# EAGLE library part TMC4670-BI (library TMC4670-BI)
Field oriented servocontrolerfor torque control,velocity control,and positioning. Encoder Engine, PWM-Engine und SPI. BGA256(17x17)
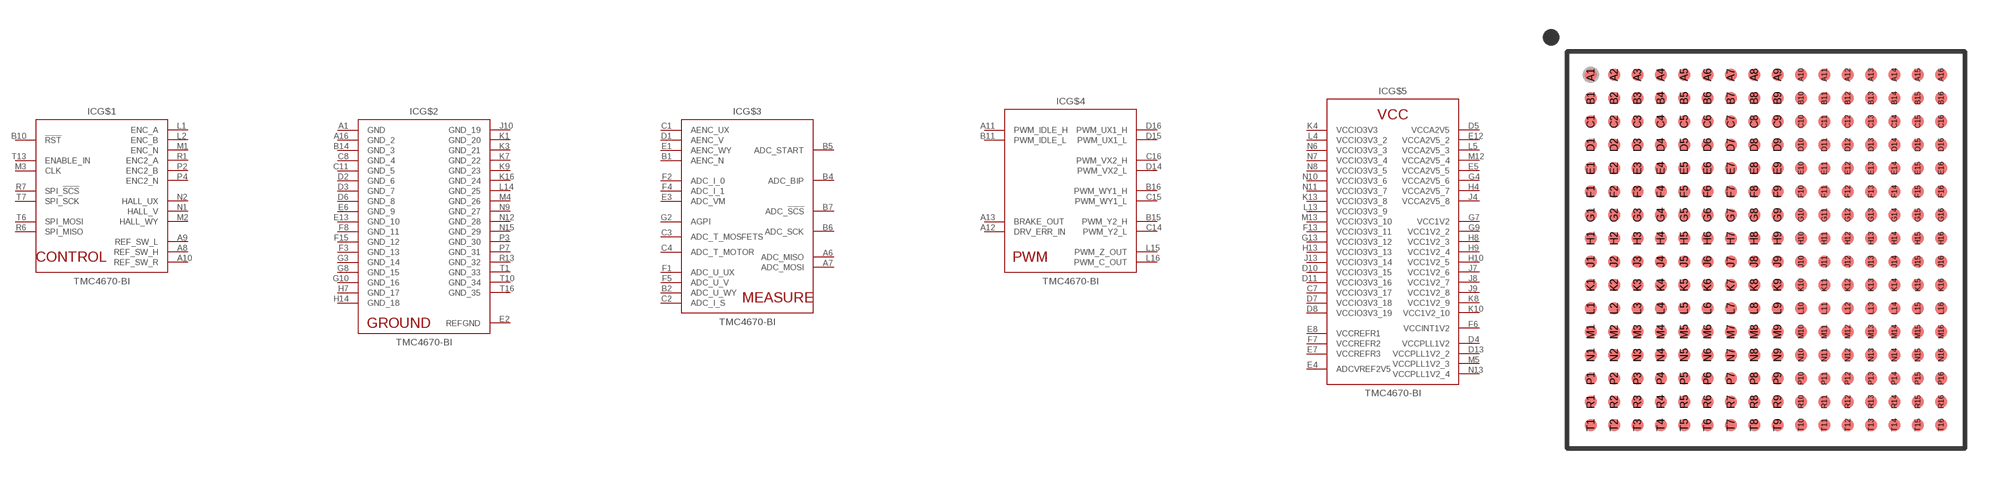
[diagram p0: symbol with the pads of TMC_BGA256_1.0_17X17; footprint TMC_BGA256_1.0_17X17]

Designator prefix IC; gates G$1=TMC4670_CONTROL G$2=TMC4670_GND G$3=TMC4670_MEASURE G$4=TMC4670_PWM G$5=TMC4670_VCC

## TMC4670-BI (DATASHEET: http://www.trinamic.com/fileadmin/assets/Products/ICs_Documents/tmc4670_datasheet.pdf; DESCRIPTION: Field oriented servocontrolerfor torque control,velocity control,and positioning_ Encoder Engine, PWM-Engine und SPI_ BGA256(17x17); GEOMETRY_HEIGHT: 2.2mm; MANUFACTURER: TRINAMIC; ORDERCODE-MANU1: TMC4670-BI; VALUE: TMC4670-BI)  [TMC_BGA256_1.0_17X17]
A1  G$2:GND  pwr
A6  G$3:ADC_MISO  out
A7  G$3:ADC_MOSI  out
A8  G$1:REF_SW_H  in
A9  G$1:REF_SW_L  in
A10  G$1:REF_SW_R  in
A11  G$4:PWM_IDLE_H  in
A12  G$4:DRV_ERR_IN  in
A13  G$4:BRAKE_OUT  out
A16  G$2:GND_2  pwr
B1  G$3:AENC_N  in
B2  G$3:ADC_U_WY  in
B4  G$3:ADC_BIP  out
B5  G$3:ADC_START  out
B6  G$3:ADC_SCK  out
B7  G$3:ADC_!SCS!  out
B10  G$1:!RST!  in
B11  G$4:PWM_IDLE_L  in
B14  G$2:GND_3  pwr
B15  G$4:PWM_Y2_H  out
B16  G$4:PWM_WY1_H  out
C1  G$3:AENC_UX  in
C2  G$3:ADC_I_S  in
C3  G$3:ADC_T_MOSFETS  in
C4  G$3:ADC_T_MOTOR  in
C7  G$5:VCCIO3V3_17  pwr
C8  G$2:GND_4  pwr
C11  G$2:GND_5  pwr
C14  G$4:PWM_Y2_L  out
C15  G$4:PWM_WY1_L  out
C16  G$4:PWM_VX2_H  out
D1  G$3:AENC_V  in
D2  G$2:GND_6  pwr
D3  G$2:GND_7  pwr
D4  G$5:VCCPLL1V2  pwr
D5  G$5:VCCA2V5  pwr
D6  G$2:GND_8  pwr
D7  G$5:VCCIO3V3_18  pwr
D8  G$5:VCCIO3V3_19  pwr
D10  G$5:VCCIO3V3_15  pwr
D11  G$5:VCCIO3V3_16  pwr
D13  G$5:VCCPLL1V2_2  pwr
D14  G$4:PWM_VX2_L  out
D15  G$4:PWM_UX1_L  out
D16  G$4:PWM_UX1_H  out
E1  G$3:AENC_WY  in
E2  G$2:REFGND  pwr
E3  G$3:ADC_VM  in
E4  G$5:ADCVREF2V5  pwr
E5  G$5:VCCA2V5_5  pwr
E6  G$2:GND_9  pwr
E7  G$5:VCCREFR3  pwr
E8  G$5:VCCREFR1  pwr
E12  G$5:VCCA2V5_2  pwr
E13  G$2:GND_10  pwr
F1  G$3:ADC_U_UX  in
F2  G$3:ADC_I_0  in
F3  G$2:GND_13  pwr
F4  G$3:ADC_I_1  in
F5  G$3:ADC_U_V  in
F6  G$5:VCCINT1V2  pwr
F7  G$5:VCCREFR2  pwr
F8  G$2:GND_11  pwr
F13  G$5:VCCIO3V3_11  pwr
F15  G$2:GND_12  pwr
G2  G$3:AGPI  in
G3  G$2:GND_14  pwr
G4  G$5:VCCA2V5_6  pwr
G7  G$5:VCC1V2  pwr
G8  G$2:GND_15  pwr
G9  G$5:VCC1V2_2  pwr
G10  G$2:GND_16  pwr
G13  G$5:VCCIO3V3_12  pwr
H4  G$5:VCCA2V5_7  pwr
H7  G$2:GND_17  pwr
H8  G$5:VCC1V2_3  pwr
H9  G$5:VCC1V2_4  pwr
H10  G$5:VCC1V2_5  pwr
H13  G$5:VCCIO3V3_13  pwr
H14  G$2:GND_18  pwr
J4  G$5:VCCA2V5_8  pwr
J7  G$5:VCC1V2_6  pwr
J8  G$5:VCC1V2_7  pwr
J9  G$5:VCC1V2_8  pwr
J10  G$2:GND_19  pwr
J13  G$5:VCCIO3V3_14  pwr
K1  G$2:GND_20  pwr
K3  G$2:GND_21  pwr
K4  G$5:VCCIO3V3  pwr
K7  G$2:GND_22  pwr
K8  G$5:VCC1V2_9  pwr
K9  G$2:GND_23  pwr
K10  G$5:VCC1V2_10  pwr
K13  G$5:VCCIO3V3_8  pwr
K16  G$2:GND_24  pwr
L1  G$1:ENC_A  in
L2  G$1:ENC_B  in
L4  G$5:VCCIO3V3_2  pwr
L5  G$5:VCCA2V5_3  pwr
L13  G$5:VCCIO3V3_9  pwr
L14  G$2:GND_25  pwr
L15  G$4:PWM_Z_OUT  out
L16  G$4:PWM_C_OUT  out
M1  G$1:ENC_N  in
M2  G$1:HALL_WY  in
M3  G$1:CLK  in
M4  G$2:GND_26  pwr
M5  G$5:VCCPLL1V2_3  pwr
M12  G$5:VCCA2V5_4  pwr
M13  G$5:VCCIO3V3_10  pwr
N1  G$1:HALL_V  in
N2  G$1:HALL_UX  in
N6  G$5:VCCIO3V3_3  pwr
N7  G$5:VCCIO3V3_4  pwr
N8  G$5:VCCIO3V3_5  pwr
N9  G$2:GND_27  pwr
N10  G$5:VCCIO3V3_6  pwr
N11  G$5:VCCIO3V3_7  pwr
N12  G$2:GND_28  pwr
N13  G$5:VCCPLL1V2_4  pwr
N15  G$2:GND_29  pwr
P2  G$1:ENC2_B  in
P3  G$2:GND_30  pwr
P4  G$1:ENC2_N  in
P7  G$2:GND_31  pwr
R1  G$1:ENC2_A  in
R6  G$1:SPI_MISO  out
R7  G$1:SPI_!SCS!  in
R13  G$2:GND_32  pwr
T1  G$2:GND_33  pwr
T6  G$1:SPI_MOSI  in
T7  G$1:SPI_SCK  in
T10  G$2:GND_34  pwr
T13  G$1:ENABLE_IN  in
T16  G$2:GND_35  pwr

## Footprint TMC_BGA256_1.0_17X17 (pad centres in mm)
smd 0.5 x 0.5: A1 -7.5,7.5; A2 -6.5,7.5; A3 -5.5,7.5; A4 -4.5,7.5; A5 -3.5,7.5; A6 -2.5,7.5; A7 -1.5,7.5; A8 -0.5,7.5; A9 0.5,7.5; A10 1.5,7.5; A11 2.5,7.5; A12 3.5,7.5; A13 4.5,7.5; A14 5.5,7.5; A15 6.5,7.5; A16 7.5,7.5; B1 -7.5,6.5; B2 -6.5,6.5; B3 -5.5,6.5; B4 -4.5,6.5; B5 -3.5,6.5; B6 -2.5,6.5; B7 -1.5,6.5; B8 -0.5,6.5; B9 0.5,6.5; B10 1.5,6.5; B11 2.5,6.5; B12 3.5,6.5; B13 4.5,6.5; B14 5.5,6.5; B15 6.5,6.5; B16 7.5,6.5; C1 -7.5,5.5; C2 -6.5,5.5; C3 -5.5,5.5; C4 -4.5,5.5; C5 -3.5,5.5; C6 -2.5,5.5; C7 -1.5,5.5; C8 -0.5,5.5; C9 0.5,5.5; C10 1.5,5.5; C11 2.5,5.5; C12 3.5,5.5; C13 4.5,5.5; C14 5.5,5.5; C15 6.5,5.5; C16 7.5,5.5; D1 -7.5,4.5; D2 -6.5,4.5; D3 -5.5,4.5; D4 -4.5,4.5; D5 -3.5,4.5; D6 -2.5,4.5; D7 -1.5,4.5; D8 -0.5,4.5; D9 0.5,4.5; D10 1.5,4.5; D11 2.5,4.5; D12 3.5,4.5; D13 4.5,4.5; D14 5.5,4.5; D15 6.5,4.5; D16 7.5,4.5; E1 -7.5,3.5; E2 -6.5,3.5; E3 -5.5,3.5; E4 -4.5,3.5; E5 -3.5,3.5; E6 -2.5,3.5; E7 -1.5,3.5; E8 -0.5,3.5; E9 0.5,3.5; E10 1.5,3.5; E11 2.5,3.5; E12 3.5,3.5; E13 4.5,3.5; E14 5.5,3.5; E15 6.5,3.5; E16 7.5,3.5; F1 -7.5,2.5; F2 -6.5,2.5; F3 -5.5,2.5; F4 -4.5,2.5; F5 -3.5,2.5; F6 -2.5,2.5; F7 -1.5,2.5; F8 -0.5,2.5; F9 0.5,2.5; F10 1.5,2.5; F11 2.5,2.5; F12 3.5,2.5; F13 4.5,2.5; F14 5.5,2.5; F15 6.5,2.5; F16 7.5,2.5; G1 -7.5,1.5; G2 -6.5,1.5; G3 -5.5,1.5; G4 -4.5,1.5; G5 -3.5,1.5; G6 -2.5,1.5; G7 -1.5,1.5; G8 -0.5,1.5; G9 0.5,1.5; G10 1.5,1.5; G11 2.5,1.5; G12 3.5,1.5; G13 4.5,1.5; G14 5.5,1.5; G15 6.5,1.5; G16 7.5,1.5; H1 -7.5,0.5; H2 -6.5,0.5; H3 -5.5,0.5; H4 -4.5,0.5; H5 -3.5,0.5; H6 -2.5,0.5; H7 -1.5,0.5; H8 -0.5,0.5; H9 0.5,0.5; H10 1.5,0.5; H11 2.5,0.5; H12 3.5,0.5; H13 4.5,0.5; H14 5.5,0.5; H15 6.5,0.5; H16 7.5,0.5; J1 -7.5,-0.5; J2 -6.5,-0.5; J3 -5.5,-0.5; J4 -4.5,-0.5; J5 -3.5,-0.5; J6 -2.5,-0.5; J7 -1.5,-0.5; J8 -0.5,-0.5; J9 0.5,-0.5; J10 1.5,-0.5; J11 2.5,-0.5; J12 3.5,-0.5; J13 4.5,-0.5; J14 5.5,-0.5; J15 6.5,-0.5; J16 7.5,-0.5; K1 -7.5,-1.5; K2 -6.5,-1.5; K3 -5.5,-1.5; K4 -4.5,-1.5; K5 -3.5,-1.5; K6 -2.5,-1.5; K7 -1.5,-1.5; K8 -0.5,-1.5; K9 0.5,-1.5; K10 1.5,-1.5; K11 2.5,-1.5; K12 3.5,-1.5; K13 4.5,-1.5; K14 5.5,-1.5; K15 6.5,-1.5; K16 7.5,-1.5; L1 -7.5,-2.5; L2 -6.5,-2.5; L3 -5.5,-2.5; L4 -4.5,-2.5; L5 -3.5,-2.5; L6 -2.5,-2.5; L7 -1.5,-2.5; L8 -0.5,-2.5; L9 0.5,-2.5; L10 1.5,-2.5; L11 2.5,-2.5; L12 3.5,-2.5; L13 4.5,-2.5; L14 5.5,-2.5; L15 6.5,-2.5; L16 7.5,-2.5; M1 -7.5,-3.5; M2 -6.5,-3.5; M3 -5.5,-3.5; M4 -4.5,-3.5; M5 -3.5,-3.5; M6 -2.5,-3.5; M7 -1.5,-3.5; M8 -0.5,-3.5; M9 0.5,-3.5; M10 1.5,-3.5; M11 2.5,-3.5; M12 3.5,-3.5; M13 4.5,-3.5; M14 5.5,-3.5; M15 6.5,-3.5; M16 7.5,-3.5; N1 -7.5,-4.5; N2 -6.5,-4.5; N3 -5.5,-4.5; N4 -4.5,-4.5; N5 -3.5,-4.5; N6 -2.5,-4.5; N7 -1.5,-4.5; N8 -0.5,-4.5; N9 0.5,-4.5; N10 1.5,-4.5; N11 2.5,-4.5; N12 3.5,-4.5; N13 4.5,-4.5; N14 5.5,-4.5; N15 6.5,-4.5; N16 7.5,-4.5; P1 -7.5,-5.5; P2 -6.5,-5.5; P3 -5.5,-5.5; P4 -4.5,-5.5; P5 -3.5,-5.5; P6 -2.5,-5.5; P7 -1.5,-5.5; P8 -0.5,-5.5; P9 0.5,-5.5; P10 1.5,-5.5; P11 2.5,-5.5; P12 3.5,-5.5; P13 4.5,-5.5; P14 5.5,-5.5; P15 6.5,-5.5; P16 7.5,-5.5; R1 -7.5,-6.5; R2 -6.5,-6.5; R3 -5.5,-6.5; R4 -4.5,-6.5; R5 -3.5,-6.5; R6 -2.5,-6.5; R7 -1.5,-6.5; R8 -0.5,-6.5; R9 0.5,-6.5; R10 1.5,-6.5; R11 2.5,-6.5; R12 3.5,-6.5; R13 4.5,-6.5; R14 5.5,-6.5; R15 6.5,-6.5; R16 7.5,-6.5; T1 -7.5,-7.5; T2 -6.5,-7.5; T3 -5.5,-7.5; T4 -4.5,-7.5; T5 -3.5,-7.5; T6 -2.5,-7.5; T7 -1.5,-7.5; T8 -0.5,-7.5; T9 0.5,-7.5; T10 1.5,-7.5; T11 2.5,-7.5; T12 3.5,-7.5; T13 4.5,-7.5; T14 5.5,-7.5; T15 6.5,-7.5; T16 7.5,-7.5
